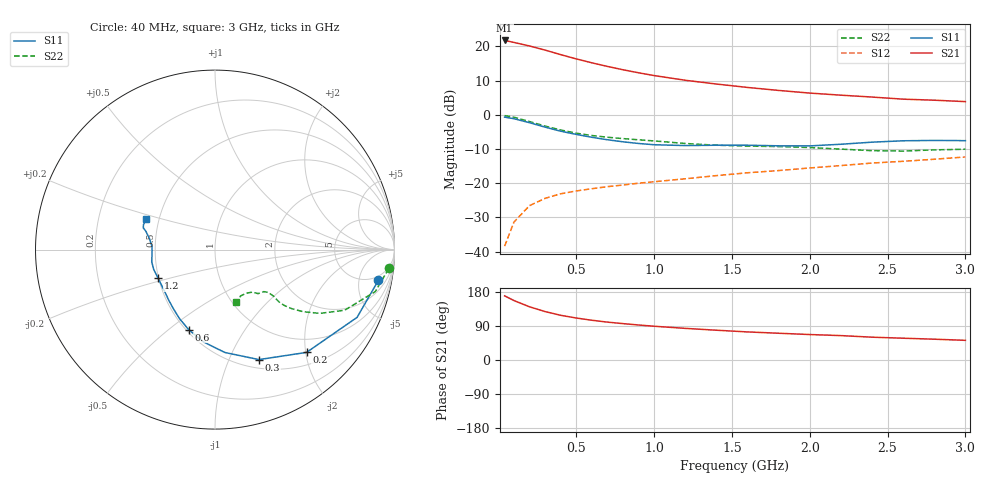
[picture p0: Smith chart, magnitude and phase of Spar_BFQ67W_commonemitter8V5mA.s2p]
! Filename:  BFQ67WH.S2P  Version:  4.0
! NXP part #: BFQ67W  Date: Jun 1994
! Bias condition: Vce=8V, Ic=5mA
#  MHz  S  MA  R  50
! Freq  S11  S21  S12  S22  !GUM [dB]
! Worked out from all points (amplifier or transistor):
!   21 points, 40 MHz to 3 GHz, reference 50 ohm
!   highest |S21| = 21.7 dB at 40 MHz (marker M1)
!   |S21| within 3 dB of that: start of sweep to 313.7 MHz
!   unconditionally stable (mu >= 1): 1.034 GHz to end of sweep
!   at 300 MHz: K = 0.44, MSG = 21.7 dB, |S12| = -24.4 dB
!   at 1 GHz: K = 0.99, MSG = 15.5 dB, |S12| = -19.6 dB
!   at 3 GHz: K = 1.06, MAG = 6.6 dB, |S12| = -12.3 dB
!   lowest NFmin = 1.50 dB at 1 GHz
!   S11 on the Smith chart (normalised r, x): 40 MHz: 3.78, -9.13; 200 MHz: 0.73, -2.02; 300 MHz: 0.60, -1.30; 600 MHz: 0.52, -0.59; 1.2 GHz: 0.50, -0.18; 3 GHz: 0.42, +0.17
40  0.926 -10.7  12.22 169.3  0.012 82.5  0.974 -6.2
100  0.877 -25.5  11.44 156.9  0.027 73.9  0.923 -14.7
200  0.767 -48.3  10.14 140.4  0.047 62.7  0.797 -25.1
300  0.66 -68.2  8.835 127.8  0.06 56.7  0.684 -31.3
400  0.576 -84.5  7.584 118.0  0.07 53.6  0.6 -35.2
500  0.517 -97.5  6.571 110.8  0.077 52.4  0.539 -37.6
600  0.469 -108.3  5.758 104.9  0.083 52.5  0.498 -38.8
700  0.432 -117.3  5.103 100.0  0.089 53.4  0.47 -39.3
800  0.403 -125.1  4.56 96.0  0.094 54.4  0.449 -39.1
900  0.381 -132.8  4.116 92.4  0.1 55.3  0.431 -38.8
1000  0.365 -140.1  3.748 89.1  0.105 56.6  0.415 -38.5
1200  0.355 -153.2  3.201 83.5  0.116 58.7  0.381 -38.8
1400  0.359 -162.3  2.818 78.6  0.129 61.0  0.359 -40.7
1600  0.359 -169.0  2.513 74.1  0.142 62.2  0.349 -43.8
1800  0.352 -175.4  2.272 70.6  0.153 64.2  0.343 -45.7
2000  0.351 177.2  2.078 67.2  0.167 65.8  0.332 -46.7
2200  0.371 170.3  1.937 64.4  0.181 67.5  0.315 -48.8
2400  0.398 165.2  1.818 60.2  0.197 68.1  0.299 -54.4
2600  0.417 163.2  1.693 57.5  0.209 68.3  0.295 -61.2
2800  0.422 160.9  1.635 54.9  0.224 69.4  0.307 -65.5
3000  0.419 156.3  1.559 51.9  0.242 69.8  0.314 -67.8
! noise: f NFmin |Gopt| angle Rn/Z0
1000  1.5  0.37  66  0.33
